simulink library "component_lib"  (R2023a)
settings: Solver=VariableStepAuto  StartTime=0.0  StopTime=10.0  RelTol=1e-3
undefined symbols (not defined in the file or in its folder): component_lib, ECCV_r, KoblenzTrier, mm, par, param_TD04, R1234yf_ph, SigIdentifier, Systems, TH0023_WP120, Thermal, V_nom
libraries: base_lib x166, $bdroot x164, simulink x2, slpidlib x1
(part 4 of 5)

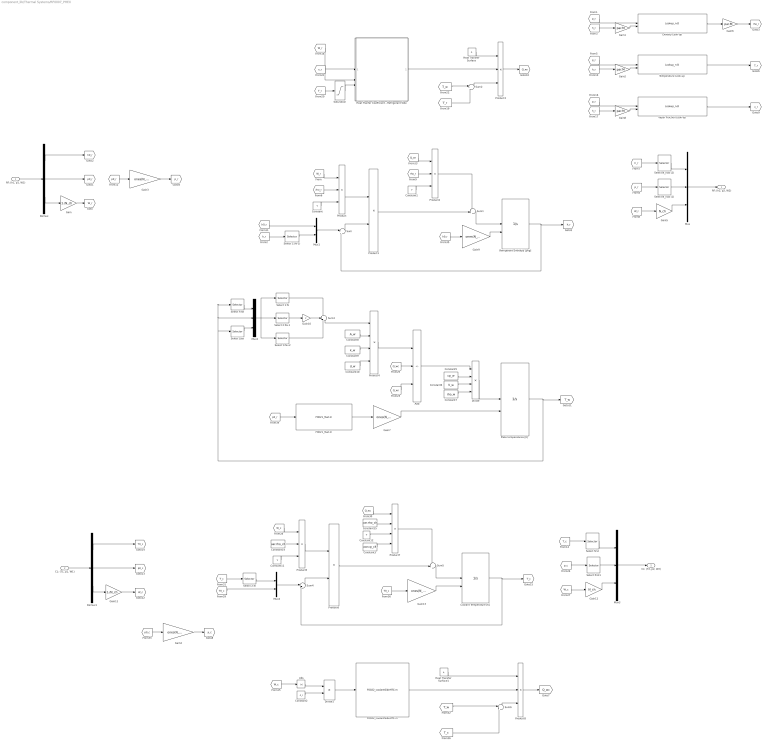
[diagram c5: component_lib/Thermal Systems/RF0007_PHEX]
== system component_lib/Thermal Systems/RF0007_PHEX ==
  "RF: (h1, p1, W1)" : Inport
  "CL: (T1, p1, W1)" : Inport  Port=2
  Abs : Abs
  Add : Sum  Inputs=+--
  Constant{,1,11..12} (4 alike) : Constant  Value=V
  Constant10 : Constant  Value=d_w
  Constant14 : Constant  Value=par.rho_clt
  Constant15 : Constant  Value=par.rho_clt
  Constant2 : Constant  Value=A_c
  Constant3 : Constant  Value=par.cp_clt
  Constant5 : Constant  Value=cp_w
  Constant6 : Constant  Value=V_w
  Constant7 : Constant  Value=rho_w
  Constant8 : Constant  Value=A_w
  Constant9 : Constant  Value=k_w
  Coolant Temperature [K] : Integrator  InitialConditionSource=external  LimitOutput=on  LowerSaturationLimit=0
  Demux : Demux  Outputs=3
  Demux1 : Demux  Outputs=3
  Density Look-up : Lookup_n-D  BreakpointsForDimension1=R1234yf_ph.p  BreakpointsForDimension2=R1234yf_ph.h  Table=R1234yf_ph.D  InternalRulePriority=Speed  RndMeth=Simplest
  Divide : Product  Inputs=*///
  Divide1 : Product  Inputs=*/
  F0021_Tsat.m : base_lib/F0021_R1234yf/F0021_Tsat.m  SystemSampleTime=-1  VariantActivationTime=update diagram  Latency=0  AutoFrameSizeCalculation=off
  F0022_coolantSideHTC.m : base_lib/F0022_heatPump/F0022_coolantSideHTC.m  SystemSampleTime=-1  VariantActivationTime=update diagram  Latency=0  AutoFrameSizeCalculation=off
  Gain : Gain  Gain=1./N_ch
  Gain{1..2,6,8} (4 alike) : Gain  Gain=par.M
  Gain10 : Gain  Gain=2
  Gain11 : Gain  Gain=1./N_ch
  Gain12 : Gain  Gain=N_ch
  Gain{3..4,7,9,13} (5 alike) : Gain  Gain=ones(N_nod,1)
  Gain5 : Gain  Gain=N_ch
  Heat Tranfer Coefficient - Refrigerant Side : Subsystem
  Heat Transfer Surface : Constant  Value=A
  Heat Transfer Surface1 : Constant  Value=A
  Mux : Mux  Inputs=3
  Mux1 : Mux  Inputs=2
  Mux2 : Mux  Inputs=3
  Mux3 : Mux  Inputs=3
  Mux4 : Mux  Inputs=2
  Plate temperatures [K] : Integrator  InitialConditionSource=external  LimitOutput=on  LowerSaturationLimit=0
  Product : Product  Inputs=*//
  Product1 : Product
  Product2 : Product  Inputs=*//
  Product3 : Product  Inputs=3
  Product4 : Product  Inputs=***/
  Product5 : Product  Inputs=*//
  Product6 : Product
  Product7 : Product  Inputs=*///
  Product8 : Product  Inputs=3
  Refrigerant Enthalpy [J/kg] : Integrator  InitialConditionSource=external  LimitOutput=on  LowerSaturationLimit=0
  Saturation : Saturate  UpperLimit=par.Tc-2  LowerLimit=0
  Select 1:(N-1) : Selector  InputPortWidth=N_nod  IndexOptions=Index vector (dialog)  Indices=[1:(N_nod-1)]  OutputSizes=1
  Select 1:N : Selector  InputPortWidth=N_nod+2  IndexOptions=Index vector (dialog)  Indices=[1:N_nod]  OutputSizes=1
  Select 2:N : Selector  InputPortWidth=N_nod  IndexOptions=Index vector (dialog)  Indices=[2:N_nod]  OutputSizes=1
  "Select 2:N+1 " : Selector  InputPortWidth=N_nod+2  IndexOptions=Index vector (dialog)  Indices=[2:(N_nod+1)]  OutputSizes=1
  Select 3:N+2 : Selector  InputPortWidth=N_nod+2  IndexOptions=Index vector (dialog)  Indices=[3:(N_nod+2)]  OutputSizes=1
  Select First : Selector  InputPortWidth=N_nod  IndexOptions=Index vector (dialog)  Indices=1  OutputSizes=1
  Select Last : Selector  InputPortWidth=N_nod  IndexOptions=Index vector (dialog)  Indices=N_nod  OutputSizes=1
  Select N_nod (1) : Selector  InputPortWidth=N_nod  IndexOptions=Index vector (dialog)  Indices=N_nod  OutputSizes=1
  Select N_nod (2) : Selector  InputPortWidth=N_nod  IndexOptions=Index vector (dialog)  Indices=N_nod  OutputSizes=1
  Select first : Selector  InputPortWidth=N_nod  IndexOptions=Index vector (dialog)  Indices=1  OutputSizes=1
  Select first1 : Selector  InputPortWidth=N_nod  IndexOptions=Index vector (dialog)  Indices=1  OutputSizes=1
  Sum{,2,4,6} (4 alike) : Sum  Inputs=|+-
  Sum1 : Sum  Inputs=++|
  Sum3 : Sum  Inputs=+-+
  Sum5 : Sum  Inputs=++|
  Temperature Look-up : Lookup_n-D  BreakpointsForDimension1=R1234yf_ph.p  BreakpointsForDimension2=R1234yf_ph.h  Table=R1234yf_ph.T  InternalRulePriority=Speed  RndMeth=Simplest
  Vapor Fraction Look-up : Lookup_n-D  BreakpointsForDimension1=R1234yf_ph.p  BreakpointsForDimension2=R1234yf_ph.h  Table=R1234yf_ph.x  InternalRulePriority=Speed  RndMeth=Simplest
  "RF: (h2, p2, W2)" : Outport
  "CL: (T2, p2, W2)" : Outport  Port=2
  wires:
  [h_r] -> Gain1/1
  Demux/2 -> [p0_r]
  "RF: (h1, p1, W1)"/1 -> Demux/1
  Mux/1 -> "RF: (h2, p2, W2)"/1
  [W_r] -> Gain5/1
  [p_r] -> Select N_nod (1)/1
  Density Look-up/1 -> Gain6/1
  Gain1/1 -> Density Look-up/2
  Gain6/1 -> [rho_r]
  Constant/1 -> Product/3
  [rho_r] -> Product/2
  [W_r] -> Product/1
  Product/1 -> Product1/1
  Sum/1 -> Product1/2
  Product1/1 -> Sum1/2
  Sum1/1 -> Refrigerant Enthalpy [J/kg]/1
  Constant1/1 -> Product2/3
  [rho_r] -> Product2/2
  Product2/1 -> Sum1/1
  Gain9/1 -> Refrigerant Enthalpy [J/kg]/2
  Refrigerant Enthalpy [J/kg]/1 -> [h_r], Sum/2
  [h_r] -> Select 1:(N-1)/1
  Select 1:(N-1)/1 -> Mux1/2
  [h0_r] -> Mux1/1
  [p_r] -> Density Look-up/1
  [p0_r] -> Gain3/1
  Gain3/1 -> [p_r]
  [h_r] -> Select N_nod (2)/1
  Select N_nod (1)/1 -> Mux/2
  Mux1/1 -> Sum/1
  [h_r] -> Gain2/1
  Gain2/1 -> Temperature Look-up/2
  [p_r] -> Temperature Look-up/1
  [Q_wr] -> Product2/1
  [h_r] -> Gain8/1
  [p_r] -> Vapor Fraction Look-up/1
  Gain8/1 -> Vapor Fraction Look-up/2
  Vapor Fraction Look-up/1 -> [x_r]
  Gain/1 -> [W_r]
  Gain7/1 -> Plate temperatures [K]/2
  Divide/1 -> Plate temperatures [K]/1
  Add/1 -> Divide/1
  Constant5/1 -> Divide/2
  Constant6/1 -> Divide/3
  Constant7/1 -> Divide/4
  [Q_wr] -> Add/3
  Plate temperatures [K]/1 -> [T_w], Select First/1, Mux2/2, Select Last/1
  Select First/1 -> Mux2/1
  Mux2/1 -> Select 3:N+2/1, "Select 2:N+1 "/1, Select 1:N/1
  Select Last/1 -> Mux2/3
  "Select 2:N+1 "/1 -> Gain10/1
  Gain10/1 -> Sum3/2
  Select 1:N/1 -> Sum3/1
  Select 3:N+2/1 -> Sum3/3
  Sum3/1 -> Product4/1
  Constant8/1 -> Product4/2
  Constant9/1 -> Product4/3
  Constant10/1 -> Product4/4
  Product4/1 -> Add/1
  [Q_wc] -> Add/2
  Gain11/1 -> [W_c]
  Demux1/2 -> [p0_c]
  "CL: (T1, p1, W1)"/1 -> Demux1/1
  [T_c] -> Select first/1
  Select first1/1 -> Mux3/2
  [W_c] -> Gain12/1
  Mux3/1 -> "CL: (T2, p2, W2)"/1
  [p_c] -> Select first1/1
  [Q_wc] -> Product7/1
  Mux4/1 -> Sum4/1
  Coolant Temperature [K]/1 -> [T_c], Sum4/2
  Product7/1 -> Sum5/1
  Gain13/1 -> Coolant Temperature [K]/2
  [T_c] -> Select 2:N/1
  Sum5/1 -> Coolant Temperature [K]/1
  Sum4/1 -> Product6/2
  Constant15/1 -> Product7/2
  Product5/1 -> Product6/1
  [W_c] -> Product5/1
  Product6/1 -> Sum5/2
  [W_r] -> Heat Tranfer Coefficient - Refrigerant Side/1(W_r [kg/s])
  [x_r] -> Heat Tranfer Coefficient - Refrigerant Side/2(x_r [-])
  [T_r] -> Saturation/1
  Heat Transfer Surface/1 -> Product3/1
  [T_w] -> Sum2/1
  Sum2/1 -> Product3/3
  [T_r] -> Sum2/2
  Product3/1 -> [Q_wr]
  Heat Tranfer Coefficient - Refrigerant Side/1(h [W/mK]) -> Product3/2
  Constant3/1 -> Product7/4
  Constant14/1 -> Product5/2
  Divide1/1 -> F0022_coolantSideHTC.m/1
  Product8/1 -> [Q_wc]
  F0022_coolantSideHTC.m/1 -> Product8/2
  Sum6/1 -> Product8/3
  [T_c] -> Sum6/2
  Temperature Look-up/1 -> [T_r]
  Gain4/1 -> [p_c]
  [p0_c] -> Gain4/1
  Saturation/1 -> Heat Tranfer Coefficient - Refrigerant Side/3(T_r [K])
  [T_w] -> Sum6/1
  Heat Transfer Surface1/1 -> Product8/1
  Constant11/1 -> Product5/3
  Constant12/1 -> Product7/3
  [T0_c] -> Mux4/2
  Select 2:N/1 -> Mux4/1
  Demux/3 -> Gain/1
  Demux/1 -> [h0_r]
  Gain5/1 -> Mux/3
  Select N_nod (2)/1 -> Mux/1
  Gain12/1 -> Mux3/3
  Select first/1 -> Mux3/1
  Demux1/3 -> Gain11/1
  Demux1/1 -> [T0_c]
  F0021_Tsat.m/1 -> Gain7/1
  [p0_r] -> F0021_Tsat.m/1
  [h0_r] -> Gain9/1
  [T0_c] -> Gain13/1
  Abs/1 -> Divide1/1
  Constant2/1 -> Divide1/2
  [W_c] -> Abs/1

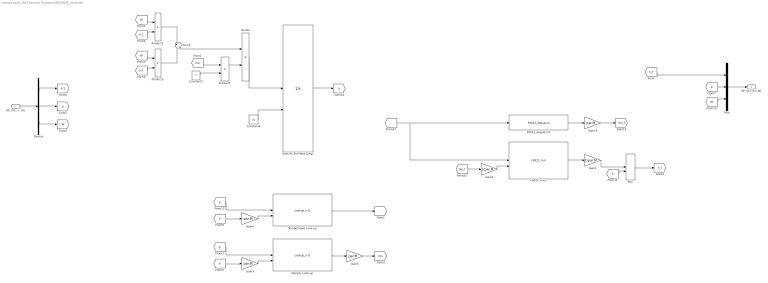
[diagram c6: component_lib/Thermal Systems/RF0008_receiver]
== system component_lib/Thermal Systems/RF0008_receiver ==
  "RF: (h1, ~, W)" : Inport
  Constant1 : Constant  Value=V
  Constant4 : Constant  Value=h0
  Demux : Demux  Outputs=3
  Density Look-up : Lookup_n-D  BreakpointsForDimension1=R1234yf_ph.p  BreakpointsForDimension2=R1234yf_ph.h  Table=R1234yf_ph.D  InternalRulePriority=Speed  RndMeth=Simplest
  Divide : Product  Inputs=*/
  F0021_dliqsat.m1 : base_lib/F0021_R1234yf/F0021_dliqsat.m  SystemSampleTime=-1  VariantActivationTime=update diagram  Latency=0  AutoFrameSizeCalculation=off
  F0021_h.m1 : base_lib/F0021_R1234yf/F0021_h.m  SystemSampleTime=-1  VariantActivationTime=update diagram  Latency=0  AutoFrameSizeCalculation=off
  Gain1 : Gain  Gain=1/par.M
  Gain{3..5,16} (4 alike) : Gain  Gain=par.M
  Gain2 : Gain  Gain=1/par.M
  Min : MinMax  Inputs=2
  Mux : Mux  Inputs=3
  Product1 : Product
  Product2 : Product
  Product3 : Product
  Specific Enthalpy [J/kg] : Integrator  InitialConditionSource=external  LimitOutput=on  LowerSaturationLimit=0
  Sum3 : Sum  Inputs=+|-
  Temperature Look-up : Lookup_n-D  BreakpointsForDimension1=R1234yf_ph.p  BreakpointsForDimension2=R1234yf_ph.h  Table=R1234yf_ph.T  InternalRulePriority=Speed  RndMeth=Simplest
  "RF: (h2, p2, W)" : Outport
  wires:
  F0021_h.m1/1 -> Gain1/1
  Gain2/1 -> F0021_h.m1/2
  [rho_f] -> Gain2/1
  [T] -> F0021_dliqsat.m1/1, F0021_h.m1/1
  F0021_dliqsat.m1/1 -> Gain16/1
  Gain16/1 -> [rho_f]
  [h_1] -> Product2/2
  [W] -> Product2/1
  Product2/1 -> Sum3/1
  [h_f] -> Product3/2
  Product3/1 -> Sum3/2
  [W] -> Product3/1
  Specific Enthalpy [J/kg]/1 -> [h]
  [h] -> Gain4/1
  Temperature Look-up/1 -> [T]
  Gain4/1 -> Temperature Look-up/2
  [p] -> Temperature Look-up/1
  Constant1/1 -> Product1/2
  [rho] -> Product1/1
  Density Look-up/1 -> Gain5/1
  Gain3/1 -> Density Look-up/2
  [p] -> Density Look-up/1
  [h] -> Gain3/1
  Gain5/1 -> [rho]
  Divide/1 -> Specific Enthalpy [J/kg]/1
  Sum3/1 -> Divide/1
  Product1/1 -> Divide/2
  Constant4/1 -> Specific Enthalpy [J/kg]/2
  Mux/1 -> "RF: (h2, p2, W)"/1
  [p] -> Mux/2
  [W] -> Mux/3
  "RF: (h1, ~, W)"/1 -> Demux/1
  Demux/1 -> [h_1]
  Demux/3 -> [W]
  [h_f] -> Mux/1
  Demux/2 -> [p]
  Min/1 -> [h_f]
  Gain1/1 -> Min/1
  [h] -> Min/2

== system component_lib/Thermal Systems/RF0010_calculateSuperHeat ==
  "RF: (h, p, W)" : Inport
  Demux : Demux  Outputs=3
  F0021_Tsat.m : base_lib/F0021_R1234yf/F0021_Tsat.m  SystemSampleTime=-1  VariantActivationTime=update diagram  Latency=0  AutoFrameSizeCalculation=off
  Gain2 : Gain  Gain=par.M
  Saturation : Saturate  UpperLimit=inf  LowerLimit=0
  Sum : Sum  Inputs=|+-
  Temperature Look-up : Lookup_n-D  BreakpointsForDimension1=R1234yf_ph.p  BreakpointsForDimension2=R1234yf_ph.h  Table=R1234yf_ph.T  InternalRulePriority=Speed  RndMeth=Simplest
  T_sup [K] : Outport
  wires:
  Demux/2 -> [p]
  Gain2/1 -> Temperature Look-up/2
  [p] -> F0021_Tsat.m/1, Temperature Look-up/1
  [h] -> Gain2/1
  Temperature Look-up/1 -> Sum/1
  F0021_Tsat.m/1 -> Sum/2
  Sum/1 -> Saturation/1
  Saturation/1 -> T_sup [K]/1
  "RF: (h, p, W)"/1 -> Demux/1
  Demux/1 -> [h]
  Demux/3 -> [W]

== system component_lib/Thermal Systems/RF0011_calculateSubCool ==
  "RF: (h, p, W)" : Inport
  Demux : Demux  Outputs=3
  F0021_Tsat.m : base_lib/F0021_R1234yf/F0021_Tsat.m  SystemSampleTime=-1  VariantActivationTime=update diagram  Latency=0  AutoFrameSizeCalculation=off
  Gain2 : Gain  Gain=par.M
  Saturation : Saturate  UpperLimit=inf  LowerLimit=0
  Sum : Sum  Inputs=|+-
  Temperature Look-up : Lookup_n-D  BreakpointsForDimension1=R1234yf_ph.p  BreakpointsForDimension2=R1234yf_ph.h  Table=R1234yf_ph.T  InternalRulePriority=Speed  RndMeth=Simplest
  T_sub [K] : Outport
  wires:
  "RF: (h, p, W)"/1 -> Demux/1
  Demux/2 -> [p]
  Gain2/1 -> Temperature Look-up/2
  [p] -> F0021_Tsat.m/1, Temperature Look-up/1
  [h] -> Gain2/1
  Sum/1 -> Saturation/1
  F0021_Tsat.m/1 -> Sum/1
  Temperature Look-up/1 -> Sum/2
  Saturation/1 -> T_sub [K]/1
  Demux/1 -> [h]
  Demux/3 -> [W]

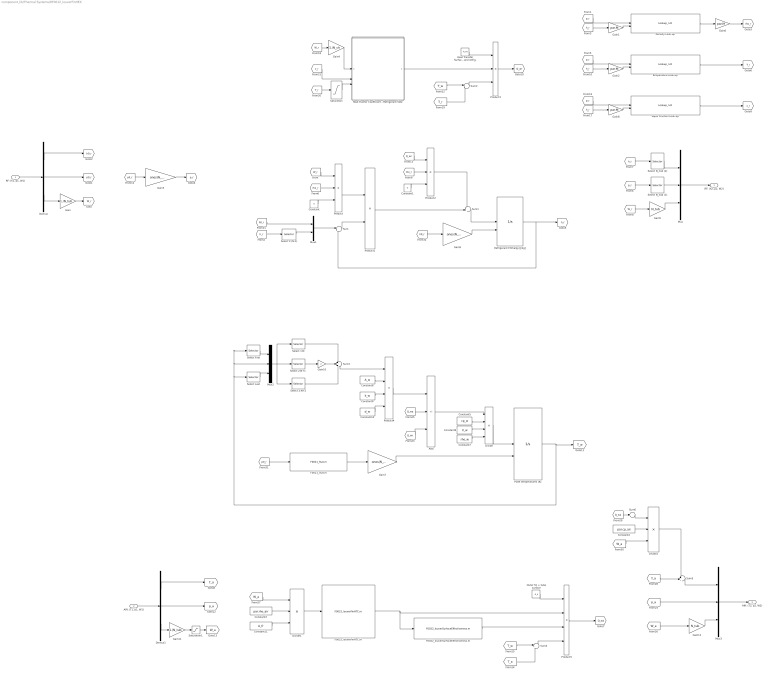
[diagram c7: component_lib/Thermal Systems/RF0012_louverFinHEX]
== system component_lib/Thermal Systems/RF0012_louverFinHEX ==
  "RF: (h1, p1, W1)" : Inport
  "AIR: (T1, p1, W1)" : Inport  Port=2
  Add : Sum  Inputs=+--
  Constant : Constant  Value=V
  Constant1 : Constant  Value=V
  Constant10 : Constant  Value=d_w
  Constant11 : Constant  Value=A_fr
  Constant2 : Constant  Value=par.cp_air
  Constant3 : Constant  Value=par.rho_air
  Constant5 : Constant  Value=cp_w
  Constant6 : Constant  Value=V_w
  Constant7 : Constant  Value=rho_w
  Constant8 : Constant  Value=A_w
  Constant9 : Constant  Value=k_w
  Demux : Demux  Outputs=3
  Demux1 : Demux  Outputs=3
  Density Look-up : Lookup_n-D  BreakpointsForDimension1=R1234yf_ph.p  BreakpointsForDimension2=R1234yf_ph.h  Table=R1234yf_ph.D  InternalRulePriority=Speed  RndMeth=Simplest
  Divide : Product  Inputs=*///
  Divide1 : Product  Inputs=*//
  Divide2 : Product  Inputs=*//
  F0021_Tsat.m : base_lib/F0021_R1234yf/F0021_Tsat.m  SystemSampleTime=-1  VariantActivationTime=update diagram  Latency=0  AutoFrameSizeCalculation=off
  F0022_louverFinHTC.m : base_lib/F0022_heatPump/F0022_louverFinHTC.m  SystemSampleTime=-1  VariantActivationTime=update diagram  Latency=0  AutoFrameSizeCalculation=off
  F0022_louverSurfaceEffectiveness.m : base_lib/F0022_heatPump/F0022_louverSurfaceEffectiveness.m  SystemSampleTime=-1  VariantActivationTime=update diagram  Latency=0  AutoFrameSizeCalculation=off
  Gain : Gain  Gain=1./N_tub
  Gain{1..2,6,8} (4 alike) : Gain  Gain=par.M
  Gain10 : Gain  Gain=2
  Gain11 : Gain  Gain=1./N_tub
  Gain12 : Gain  Gain=N_tub
  Gain3 : Gain  Gain=ones(N_nod,1)
  Gain4 : Gain  Gain=1./N_ch
  Gain5 : Gain  Gain=N_tub
  Gain7 : Gain  Gain=ones(N_nod,1)
  Gain9 : Gain  Gain=ones(N_nod,1)
  Heat Tranfer Coefficient - Refrigerant Side : Subsystem
  Heat Transfer Surface between wall and refrig. : Constant  Value=A_wr
  Mux : Mux  Inputs=3
  Mux1 : Mux  Inputs=2
  Mux2 : Mux  Inputs=3
  Mux3 : Mux  Inputs=3
  Outer fin + tube surface : Constant  Value=A_o
  Plate temperatures [K] : Integrator  InitialConditionSource=external  LimitOutput=on  LowerSaturationLimit=0
  Product : Product  Inputs=*//
  Product1 : Product
  Product2 : Product  Inputs=*//
  Product3 : Product  Inputs=3
  Product4 : Product  Inputs=***/
  Product5 : Product  Inputs=4
  Refrigerant Enthalpy [J/kg] : Integrator  InitialConditionSource=external  LimitOutput=on  LowerSaturationLimit=0
  Saturation : Saturate  UpperLimit=par.Tc-2  LowerLimit=0
  Saturation1 : Saturate  UpperLimit=inf  LowerLimit=1e-5
  Select 1:(N-1) : Selector  InputPortWidth=N_nod  IndexOptions=Index vector (dialog)  Indices=[1:(N_nod-1)]  OutputSizes=1
  Select 1:N : Selector  InputPortWidth=N_nod+2  IndexOptions=Index vector (dialog)  Indices=[1:N_nod]  OutputSizes=1
  "Select 2:N+1 " : Selector  InputPortWidth=N_nod+2  IndexOptions=Index vector (dialog)  Indices=[2:(N_nod+1)]  OutputSizes=1
  Select 3:N+2 : Selector  InputPortWidth=N_nod+2  IndexOptions=Index vector (dialog)  Indices=[3:(N_nod+2)]  OutputSizes=1
  Select First : Selector  InputPortWidth=N_nod  IndexOptions=Index vector (dialog)  Indices=1  OutputSizes=1
  Select Last : Selector  InputPortWidth=N_nod  IndexOptions=Index vector (dialog)  Indices=N_nod  OutputSizes=1
  Select N_nod (1) : Selector  InputPortWidth=N_nod  IndexOptions=Index vector (dialog)  Indices=N_nod  OutputSizes=1
  Select N_nod (2) : Selector  InputPortWidth=N_nod  IndexOptions=Index vector (dialog)  Indices=N_nod  OutputSizes=1
  Sum : Sum  Inputs=|+-
  Sum1 : Sum  Inputs=++|
  Sum2 : Sum  Inputs=|+-
  Sum3 : Sum  Inputs=+-+
  Sum4 : Sum  Inputs=|+-
  Sum5 : Sum  Inputs=++|
  Sum6 : Sum  Inputs=+
  Temperature Look-up : Lookup_n-D  BreakpointsForDimension1=R1234yf_ph.p  BreakpointsForDimension2=R1234yf_ph.h  Table=R1234yf_ph.T  InternalRulePriority=Speed  RndMeth=Simplest
  Vapor Fraction Look-up : Lookup_n-D  BreakpointsForDimension1=R1234yf_ph.p  BreakpointsForDimension2=R1234yf_ph.h  Table=R1234yf_ph.x  InternalRulePriority=Speed  RndMeth=Simplest
  "RF: (h2, p2, W2)" : Outport
  "AIR: (T2, p2, W2)" : Outport  Port=2
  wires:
  Select N_nod (2)/1 -> Mux/1
  Gain5/1 -> Mux/3
  Demux/1 -> [h0_r]
  Demux/3 -> Gain/1
  Saturation/1 -> Heat Tranfer Coefficient - Refrigerant Side/3(T_r [K])
  Temperature Look-up/1 -> [T_r]
  Heat Tranfer Coefficient - Refrigerant Side/1(h [W/mK]) -> Product3/2
  Product3/1 -> [Q_wr]
  [T_r] -> Sum2/2
  Sum2/1 -> Product3/3
  [T_w] -> Sum2/1
  Heat Transfer Surface between wall and refrig./1 -> Product3/1
  [T_r] -> Saturation/1
  [x_r] -> Heat Tranfer Coefficient - Refrigerant Side/2(x_r [-])
  Mux3/1 -> "AIR: (T2, p2, W2)"/1
  "AIR: (T1, p1, W1)"/1 -> Demux1/1
  [Q_wa] -> Add/2
  Product4/1 -> Add/1
  Constant10/1 -> Product4/4
  Constant8/1 -> Product4/2
  Sum3/1 -> Product4/1
  Select 3:N+2/1 -> Sum3/3
  Select 1:N/1 -> Sum3/1
  Gain10/1 -> Sum3/2
  "Select 2:N+1 "/1 -> Gain10/1
  Select Last/1 -> Mux2/3
  Mux2/1 -> Select 1:N/1, "Select 2:N+1 "/1, Select 3:N+2/1
  Select First/1 -> Mux2/1
  Plate temperatures [K]/1 -> Mux2/2, Select First/1, Select Last/1, [T_w]
  [Q_wr] -> Add/3
  Constant7/1 -> Divide/4
  Constant6/1 -> Divide/3
  Constant5/1 -> Divide/2
  Add/1 -> Divide/1
  Divide/1 -> Plate temperatures [K]/1
  Gain7/1 -> Plate temperatures [K]/2
  Gain/1 -> [W_r]
  Vapor Fraction Look-up/1 -> [x_r]
  Gain8/1 -> Vapor Fraction Look-up/2
  [p_r] -> Vapor Fraction Look-up/1
  [h_r] -> Gain8/1
  [Q_wr] -> Product2/1
  [p_r] -> Temperature Look-up/1
  Gain2/1 -> Temperature Look-up/2
  [h_r] -> Gain2/1
  Mux1/1 -> Sum/1
  Select N_nod (1)/1 -> Mux/2
  [h_r] -> Select N_nod (2)/1
  Gain3/1 -> [p_r]
  [p0_r] -> Gain3/1
  [p_r] -> Density Look-up/1
  [h0_r] -> Mux1/1
  Select 1:(N-1)/1 -> Mux1/2
  [h_r] -> Select 1:(N-1)/1
  Refrigerant Enthalpy [J/kg]/1 -> Sum/2, [h_r]
  Gain9/1 -> Refrigerant Enthalpy [J/kg]/2
  Product2/1 -> Sum1/1
  [rho_r] -> Product2/2
  Constant1/1 -> Product2/3
  Sum1/1 -> Refrigerant Enthalpy [J/kg]/1
  Product1/1 -> Sum1/2
  Sum/1 -> Product1/2
  Product/1 -> Product1/1
  [W_r] -> Product/1
  [rho_r] -> Product/2
  Constant/1 -> Product/3
  Gain6/1 -> [rho_r]
  Gain1/1 -> Density Look-up/2
  Density Look-up/1 -> Gain6/1
  [p_r] -> Select N_nod (1)/1
  [W_r] -> Gain5/1
  Mux/1 -> "RF: (h2, p2, W2)"/1
  "RF: (h1, p1, W1)"/1 -> Demux/1
  Demux/2 -> [p0_r]
  [h_r] -> Gain1/1
  F0022_louverFinHTC.m/1 -> Product5/2, F0022_louverSurfaceEffectiveness.m/1
  Divide1/1 -> F0022_louverFinHTC.m/1
  Constant3/1 -> Divide1/2
  Constant11/1 -> Divide1/3
  Product5/1 -> [Q_wa]
  [T_w] -> Sum4/1
  Outer fin + tube surface/1 -> Product5/1
  [T_a] -> Sum4/2
  Sum4/1 -> Product5/4
  F0022_louverSurfaceEffectiveness.m/1 -> Product5/3
  Demux1/1 -> [T_a]
  Demux1/2 -> [p_a]
  [p_a] -> Mux3/2
  Demux1/3 -> Gain11/1
  [W_a] -> Divide1/1
  [W_r] -> Gain4/1
  Gain4/1 -> Heat Tranfer Coefficient - Refrigerant Side/1(W_r [kg/s])
  [p0_r] -> F0021_Tsat.m/1
  F0021_Tsat.m/1 -> Gain7/1
  [h0_r] -> Gain9/1
  Constant9/1 -> Product4/3
  Gain12/1 -> Mux3/3
  Gain11/1 -> Saturation1/1
  [W_a] -> Gain12/1
  [T_a] -> Sum5/2
  Sum5/1 -> Mux3/1
  [Q_wa] -> Sum6/1
  Sum6/1 -> Divide2/1
  Constant2/1 -> Divide2/2
  [W_a] -> Divide2/3
  Divide2/1 -> Sum5/1
  Saturation1/1 -> [W_a]

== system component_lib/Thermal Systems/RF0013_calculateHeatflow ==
  "RF: (h1, p1, W1)" : Inport
  "RF: (h2, p2, W2)" : Inport  Port=2
  Demux : Demux  Outputs=3
  Demux1 : Demux  Outputs=3
  Product : Product
  Product1 : Product
  Sum : Sum  Inputs=|+-
  Terminator : Terminator
  Terminator1 : Terminator
  Q [J/s] : Outport
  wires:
  "RF: (h1, p1, W1)"/1 -> Demux/1
  "RF: (h2, p2, W2)"/1 -> Demux1/1
  Sum/1 -> Q [J/s]/1
  Demux/2 -> Terminator/1
  Demux1/2 -> Terminator1/1
  Demux/1 -> Product/1
  Demux/3 -> Product/2
  Demux1/1 -> Product1/1
  Demux1/3 -> Product1/2
  Product1/1 -> Sum/1
  Product/1 -> Sum/2

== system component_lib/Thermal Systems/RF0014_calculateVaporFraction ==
  "RF: (h, p, W)" : Inport
  Demux : Demux  Outputs=3
  Gain2 : Gain  Gain=par.M
  Vapor Fraction Look-up : Lookup_n-D  BreakpointsForDimension1=R1234yf_ph.p  BreakpointsForDimension2=R1234yf_ph.h  Table=R1234yf_ph.x  InternalRulePriority=Speed  RndMeth=Simplest
  x [-] : Outport
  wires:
  Demux/2 -> [p]
  Gain2/1 -> Vapor Fraction Look-up/2
  [p] -> Vapor Fraction Look-up/1
  [h] -> Gain2/1
  Vapor Fraction Look-up/1 -> x [-]/1
  "RF: (h, p, W)"/1 -> Demux/1
  Demux/1 -> [h]
  Demux/3 -> [W]

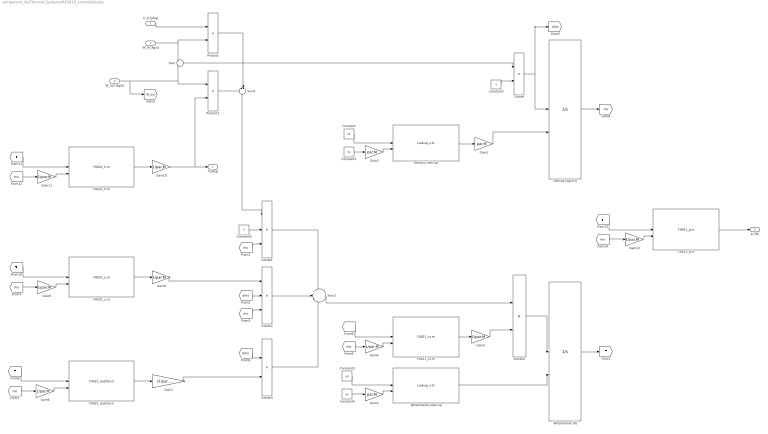
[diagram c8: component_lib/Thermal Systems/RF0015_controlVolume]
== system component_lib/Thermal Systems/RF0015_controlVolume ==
  h_in [J/kg] : Inport
  W_in [kg/s] : Inport  Port=2
  W_out [kg/s] : Inport  Port=3
  Constant : Constant  Value=p0
  Constant1 : Constant  Value=h0
  Constant2 : Constant  Value=V
  Constant3 : Constant  Value=p0
  Constant4 : Constant  Value=h0
  Constant5 : Constant  Value=V
  Density Look-up : Lookup_n-D  BreakpointsForDimension1=R1234yf_ph.p  BreakpointsForDimension2=R1234yf_ph.h  Table=R1234yf_ph.D  InternalRulePriority=Speed  RndMeth=Simplest
  Density [kg/m3] : Integrator  InitialConditionSource=external  LimitOutput=on  LowerSaturationLimit=0
  Divide : Product  Inputs=*/
  Divide1 : Product  Inputs=*//
  Divide2 : Product  Inputs=**/
  Divide3 : Product  Inputs=**
  Divide4 : Product  Inputs=*/
  F0021_cv.m : base_lib/F0021_R1234yf/F0021_cv.m  SystemSampleTime=-1  VariantActivationTime=update diagram  Latency=0  AutoFrameSizeCalculation=off
  F0021_dudrho.m : base_lib/F0021_R1234yf/F0021_dudrho.m  SystemSampleTime=-1  VariantActivationTime=update diagram  Latency=0  AutoFrameSizeCalculation=off
  F0021_h.m : base_lib/F0021_R1234yf/F0021_h.m  SystemSampleTime=-1  VariantActivationTime=update diagram  Latency=0  AutoFrameSizeCalculation=off
  F0021_p.m : base_lib/F0021_R1234yf/F0021_p.m  SystemSampleTime=-1  VariantActivationTime=update diagram  Latency=0  AutoFrameSizeCalculation=off
  F0021_u.m : base_lib/F0021_R1234yf/F0021_u.m  SystemSampleTime=-1  VariantActivationTime=update diagram  Latency=0  AutoFrameSizeCalculation=off
  Gain1 : Gain  Gain=par.M
  Gain{4..6,8..12} (8 alike) : Gain  Gain=1/par.M
  Gain2 : Gain  Gain=par.M
  Gain3 : Gain  Gain=par.M
  Gain7 : Gain  Gain=(1/par.M).^2
  Product : Product
  Product1 : Product
  Sum : Sum  Inputs=+|-
  Sum1 : Sum  Inputs=-+|
  Sum2 : Sum  Inputs=+--
  Temperature Look-up : Lookup_n-D  BreakpointsForDimension1=R1234yf_ph.p  BreakpointsForDimension2=R1234yf_ph.h  Table=R1234yf_ph.T  InternalRulePriority=Speed  RndMeth=Simplest
  Temperature [K] : Integrator  InitialConditionSource=external  LimitOutput=on  LowerSaturationLimit=0
  h [J/kg] : Outport
  p [Pa] : Outport  Port=2
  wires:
  Density Look-up/1 -> Gain1/1
  Gain1/1 -> Density [kg/m3]/2
  Constant/1 -> Density Look-up/1
  Gain3/1 -> Density Look-up/2
  Constant1/1 -> Gain3/1
  Divide/1 -> Density [kg/m3]/1, [drho]
  Constant2/1 -> Divide/2
  Density [kg/m3]/1 -> [rho]
  Sum/1 -> Divide/1
  W_out [kg/s]/1 -> [W_out], Product1/1, Sum/2
  Temperature Look-up/1 -> Temperature [K]/2
  Gain2/1 -> Temperature Look-up/2
  Constant4/1 -> Gain2/1
  Constant3/1 -> Temperature Look-up/1
  Temperature [K]/1 -> [T]
  W_in [kg/s]/1 -> Product/2, Sum/1
  h_in [J/kg]/1 -> Product/1
  Gain10/1 -> h [J/kg]/1, Product1/2
  Product/1 -> Sum1/2
  Product1/1 -> Sum1/1
  Sum1/1 -> Divide1/1
  Constant5/1 -> Divide1/2
  [rho] -> Divide1/3
  [rho] -> Divide2/3
  [drho] -> Divide2/2
  Gain9/1 -> Divide2/1
  [rho] -> Gain4/1
  Gain4/1 -> F0021_cv.m/2
  F0021_cv.m/1 -> Gain5/1
  [T] -> F0021_cv.m/1
  Divide4/1 -> Temperature [K]/1
  Gain5/1 -> Divide4/2
  Sum2/1 -> Divide4/1
  Divide1/1 -> Sum2/1
  Divide2/1 -> Sum2/2
  Divide3/1 -> Sum2/3
  [rho] -> Gain6/1
  Gain6/1 -> F0021_dudrho.m/2
  [T] -> F0021_dudrho.m/1
  [drho] -> Divide3/1
  F0021_dudrho.m/1 -> Gain7/1
  Gain7/1 -> Divide3/2
  [T] -> F0021_u.m/1
  [rho] -> Gain8/1
  Gain8/1 -> F0021_u.m/2
  F0021_u.m/1 -> Gain9/1
  F0021_h.m/1 -> Gain10/1
  [rho] -> Gain11/1
  Gain11/1 -> F0021_h.m/2
  [T] -> F0021_h.m/1
  F0021_p.m/1 -> p [Pa]/1
  [rho] -> Gain12/1
  Gain12/1 -> F0021_p.m/2
  [T] -> F0021_p.m/1

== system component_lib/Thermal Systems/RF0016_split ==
  "RF A: (h, p, W)" : Inport
  split [-] : Inport  Port=2
  Constant : Constant
  Demux : Demux  Outputs=3
  Mux : Mux  Inputs=3
  Mux1 : Mux  Inputs=3
  Product : Product
  Product1 : Product
  Sum : Sum  Inputs=-+|
  "RF B: (h, p, Wb)" : Outport
  "RF C: (h, p, Wc)" : Outport  Port=2
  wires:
  "RF A: (h, p, W)"/1 -> Demux/1
  Mux/1 -> "RF B: (h, p, Wb)"/1
  Mux1/1 -> "RF C: (h, p, Wc)"/1
  Demux/3 -> [W]
  Demux/2 -> [p]
  Demux/1 -> [h]
  split [-]/1 -> Sum/1, Product/2
  [W] -> Product/1
  Constant/1 -> Sum/2
  Sum/1 -> Product1/2
  [W] -> Product1/1
  Product/1 -> Mux/3
  [p] -> Mux/2
  [p] -> Mux1/2
  [h] -> Mux/1
  [h] -> Mux1/1
  Product1/1 -> Mux1/3

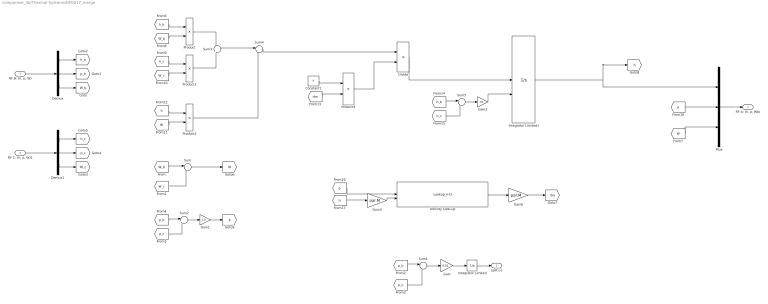
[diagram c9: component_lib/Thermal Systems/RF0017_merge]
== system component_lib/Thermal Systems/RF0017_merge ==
  "RF B: (h, p, W)" : Inport
  "RF C: (h, p, W)1" : Inport  Port=2
  Constant1 : Constant  Value=V
  Demux : Demux  Outputs=3
  Demux1 : Demux  Outputs=3
  Density Look-up : Lookup_n-D  BreakpointsForDimension1=R1234yf_ph.p  BreakpointsForDimension2=R1234yf_ph.h  Table=R1234yf_ph.D  InternalRulePriority=Speed  RndMeth=Simplest
  Divide : Product  Inputs=*/
  Gain : Gain  Gain=0.01
  Gain1 : Gain  Gain=1/2
  Gain2 : Gain  Gain=1/2
  Gain3 : Gain  Gain=par.M
  Gain6 : Gain  Gain=par.M
  Integrator Limited : Integrator  InitialCondition=0.5  LimitOutput=on  UpperSaturationLimit=1  LowerSaturationLimit=0
  Integrator Limited1 : Integrator  InitialConditionSource=external  InitialCondition=0.5  LimitOutput=on  LowerSaturationLimit=0
  Mux : Mux  Inputs=3
  Product{,1..2,4} (4 alike) : Product
  Sum : Sum  Inputs=|++
  Sum1 : Sum  Inputs=|+-
  Sum2 : Sum  Inputs=|++
  Sum3 : Sum  Inputs=+|+
  Sum4 : Sum  Inputs=|+-
  Sum5 : Sum  Inputs=|++
  "RF A: (h, p, Wb)" : Outport
  split [-] : Outport  Port=2
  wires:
  "RF B: (h, p, W)"/1 -> Demux/1
  Mux/1 -> "RF A: (h, p, Wb)"/1
  Demux/3 -> [W_b]
  Demux/2 -> [p_b]
  Demux/1 -> [h_b]
  Sum2/1 -> Gain1/1
  Demux1/1 -> [h_c]
  Demux1/3 -> [W_c]
  Demux1/2 -> [p_c]
  "RF C: (h, p, W)1"/1 -> Demux1/1
  [W_b] -> Sum/1
  [W_c] -> Sum/2
  [p_c] -> Sum1/2
  [p_b] -> Sum1/1
  Gain/1 -> Integrator Limited/1
  Sum1/1 -> Gain/1
  Integrator Limited/1 -> split [-]/1
  [p_b] -> Sum2/1
  [p_c] -> Sum2/2
  [h_b] -> Product/1
  [W_b] -> Product/2
  [W_c] -> Product1/2
  [h_c] -> Product1/1
  Product/1 -> Sum3/1
  Product1/1 -> Sum3/2
  Sum3/1 -> Sum4/1
  Sum/1 -> [W]
  [h] -> Product2/1
  [W] -> Product2/2
  [W] -> Mux/3
  Product2/1 -> Sum4/2
  Constant1/1 -> Product4/1
  [rho] -> Product4/2
  [h_b] -> Sum5/1
  [h_c] -> Sum5/2
  Sum5/1 -> Gain2/1
  Gain2/1 -> Integrator Limited1/2
  Divide/1 -> Integrator Limited1/1
  Sum4/1 -> Divide/1
  Product4/1 -> Divide/2
  Integrator Limited1/1 -> [h], Mux/1
  Density Look-up/1 -> Gain6/1
  [h] -> Gain3/1
  Gain3/1 -> Density Look-up/2
  Gain6/1 -> [rho]
  [p] -> Density Look-up/1
  Gain1/1 -> [p]
  [p] -> Mux/2

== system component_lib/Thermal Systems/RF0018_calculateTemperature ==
  "RF: (h, p, W)" : Inport
  Demux : Demux  Outputs=3
  Gain2 : Gain  Gain=par.M
  Temperature Look-up : Lookup_n-D  BreakpointsForDimension1=R1234yf_ph.p  BreakpointsForDimension2=R1234yf_ph.h  Table=R1234yf_ph.T  InternalRulePriority=Speed  RndMeth=Simplest
  T [K] : Outport
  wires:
  "RF: (h, p, W)"/1 -> Demux/1
  Demux/2 -> [p]
  Gain2/1 -> Temperature Look-up/2
  [p] -> Temperature Look-up/1
  [h] -> Gain2/1
  Temperature Look-up/1 -> T [K]/1
  Demux/1 -> [h]
  Demux/3 -> [W]

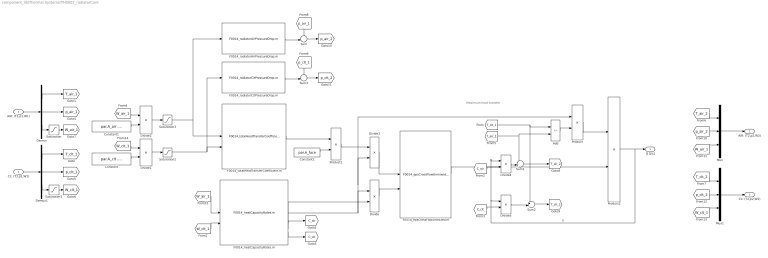
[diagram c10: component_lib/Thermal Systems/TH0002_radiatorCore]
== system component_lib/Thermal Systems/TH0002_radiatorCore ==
  note: Maximum heat transfer
  AIR: (T1,p1,W1) : Inport
  CL: (T1,p1,W1) : Inport  Port=2
  Add : Sum  Inputs=+-
  Constant : Constant  Value=par.A_clt .* par.rho_clt
  Constant1 : Constant  Value=par.A_air .* par.rho_air
  Constant2 : Constant  Value=par.A_face
  Demux : Demux  Outputs=3
  Demux1 : Demux  Outputs=3
  Divide{,1..5} (6 alike) : Product  Inputs=*/
  F0014_epsCrossFlowUnmixed.m : base_lib/F0014_titanXradiator/F0014_epsCrossFlowUnmixed.m  SystemSampleTime=-1  VariantActivationTime=update diagram  Latency=0  AutoFrameSizeCalculation=off
  F0014_heatCapacityRates.m : base_lib/F0014_titanXradiator/F0014_heatCapacityRates.m  SystemSampleTime=-1  VariantActivationTime=update diagram  Latency=0  AutoFrameSizeCalculation=off
  F0014_radiatorAirPressureDrop.m : base_lib/F0014_titanXradiator/F0014_radiatorAirPressureDrop.m  SystemSampleTime=-1  VariantActivationTime=update diagram  Latency=0  AutoFrameSizeCalculation=off
  F0014_radiatorCltPressureDrop.m : base_lib/F0014_titanXradiator/F0014_radiatorCltPressureDrop.m  SystemSampleTime=-1  VariantActivationTime=update diagram  Latency=0  AutoFrameSizeCalculation=off
  F0014_totalHeatTransferCoefficient.m : base_lib/F0014_titanXradiator/F0014_totalHeatTransferCoefficient.m  SystemSampleTime=-1  VariantActivationTime=update diagram  Latency=0  AutoFrameSizeCalculation=off
  Mux : Mux  Inputs=3
  Mux1 : Mux  Inputs=3
  Product : Product
  Product1 : Product
  Product2 : Product
  Saturation : Saturate  UpperLimit=inf  LowerLimit=1e-5
  Saturation1 : Saturate  UpperLimit=inf  LowerLimit=1e-5
  Saturation2 : Saturate  UpperLimit=inf  LowerLimit=1e-3
  Saturation3 : Saturate  UpperLimit=inf  LowerLimit=1e-3
  Sum : Sum  Inputs=+-|
  Sum1 : Sum  Inputs=++|
  Sum2 : Sum  Inputs=+-|
  Sum3 : Sum  Inputs=+-|
  Q [J/s] : Outport
  AIR: (T2,p2,W2) : Outport  Port=2
  CL: (T2,p2,W2) : Outport  Port=3
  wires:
  F0014_heatCapacityRates.m/2 -> Divide/2
  F0014_heatCapacityRates.m/1 -> Product/1, Divide3/2, Divide/1
  Divide/1 -> F0014_epsCrossFlowUnmixed.m/2
  Constant/1 -> Divide1/2
  Divide1/1 -> Saturation2/1
  [W_air_1] -> Divide2/1
  Constant1/1 -> Divide2/2
  Divide2/1 -> Saturation3/1
  F0014_totalHeatTransferCoefficient.m/1 -> Product1/1
  Constant2/1 -> Product1/2
  Product1/1 -> Divide3/1
  Divide3/1 -> F0014_epsCrossFlowUnmixed.m/1
  F0014_epsCrossFlowUnmixed.m/1 -> Product2/2
  Add/1 -> Product/2
  Product2/1 -> Q [J/s]/1, Divide4/1, Divide5/1  "Q"
  [T_clt_1] -> Sum2/1, Add/1
  Product/1 -> Product2/1
  F0014_heatCapacityRates.m/3 -> [C_air]
  F0014_heatCapacityRates.m/4 -> [C_clt]
  [T_air_1] -> Add/2, Sum1/1
  Divide4/1 -> Sum1/2
  [C_air] -> Divide4/2
  [C_clt] -> Divide5/2
  Divide5/1 -> Sum2/2
  AIR: (T1,p1,W1)/1 -> Demux/1
  CL: (T1,p1,W1)/1 -> Demux1/1
  Demux1/1 -> [T_clt_1]
  Demux/1 -> [T_air_1]
  Demux/2 -> [p_air_1]
  Demux1/2 -> [p_clt_1]
  Sum1/1 -> [T_air_2]
  Sum2/1 -> [T_clt_2]
  Mux/1 -> AIR: (T2,p2,W2)/1
  [p_air_1] -> Sum/1
  F0014_radiatorAirPressureDrop.m/1 -> Sum/2
  Sum/1 -> [p_air_2]
  Sum3/1 -> [p_clt_2]
  F0014_radiatorCltPressureDrop.m/1 -> Sum3/2
  [p_clt_1] -> Sum3/1
  [T_clt_2] -> Mux1/1
  [T_air_2] -> Mux/1
  [p_air_2] -> Mux/2
  [W_air_1] -> Mux/3
  [p_clt_2] -> Mux1/2
  [W_clt_1] -> Mux1/3
  Mux1/1 -> CL: (T2,p2,W2)/1
  Demux1/3 -> Saturation1/1
  Saturation1/1 -> [W_clt_1]
  Demux/3 -> Saturation/1
  Saturation/1 -> [W_air_1]
  [W_clt_1] -> F0014_heatCapacityRates.m/2
  [W_clt_1] -> Divide1/1
  [W_air_1] -> F0014_heatCapacityRates.m/1
  Saturation2/1 -> F0014_radiatorCltPressureDrop.m/1, F0014_totalHeatTransferCoefficient.m/2
  Saturation3/1 -> F0014_radiatorAirPressureDrop.m/1, F0014_totalHeatTransferCoefficient.m/1

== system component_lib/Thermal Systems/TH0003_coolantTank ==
  CL: (T1,p1,W1) : Inport
  Coolant density : Constant  Value=par.rho_clt
  Coolant density1 : Constant  Value=par.rho_clt
  Demux1 : Demux  Outputs=3
  Divide : Product  Inputs=*/
  F0014_tankPressureDrop.m : base_lib/F0014_titanXradiator/F0014_tankPressureDrop.m  SystemSampleTime=-1  VariantActivationTime=update diagram  Latency=0  AutoFrameSizeCalculation=off
  Integrator : Integrator  InitialCondition=T_0
  Mixing/Mass factor - empirical : Gain  Gain=3
  Mux1 : Mux  Inputs=3
  Product : Product
  Product1 : Product
  Product3 : Product  Inputs=*/
  Product5 : Product  Inputs=*/
  Subtract : Sum  Inputs=+-
  Sum : Sum  Inputs=|+-
  Tank volume : Constant  Value=par.V
  connector inlet area : Constant  Value=par.A_con
  CL: (T2,p2,W2) : Outport
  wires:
  CL: (T1,p1,W1)/1 -> Demux1/1
  Demux1/3 -> [W_clt_1]
  Demux1/1 -> [T_clt_1]
  Demux1/2 -> [p_clt_1]
  Mux1/1 -> CL: (T2,p2,W2)/1
  [p_clt_2] -> Mux1/2
  [W_clt_1] -> Mux1/3
  [T_clt_2] -> Mux1/1
  Tank volume/1 -> Mixing/Mass factor - empirical/1
  [W_clt_1] -> Product5/1
  [p_clt_1] -> Sum/1
  [T_clt_1] -> Subtract/1
  [W_clt_1] -> Product1/2
  Subtract/1 -> Product1/1
  Integrator/1 -> [T_clt_2], Subtract/2
  Coolant density/1 -> Product5/2
  Mixing/Mass factor - empirical/1 -> Product/1
  Product/1 -> Divide/2
  Product1/1 -> Divide/1
  connector inlet area/1 -> Product3/2
  Sum/1 -> [p_clt_2]
  Product5/1 -> Product3/1
  Divide/1 -> Integrator/1
  F0014_tankPressureDrop.m/1 -> Sum/2
  Product3/1 -> F0014_tankPressureDrop.m/1  "v"
  Coolant density1/1 -> Product/2

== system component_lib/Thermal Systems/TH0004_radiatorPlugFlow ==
  CL: (T1,p1,W1) : Inport
  Demux1 : Demux  Outputs=3
  F0014_coreFlowDelay.m : base_lib/F0014_titanXradiator/F0014_coreFlowDelay.m  SystemSampleTime=-1  VariantActivationTime=update diagram  Latency=0  AutoFrameSizeCalculation=off
  Mux1 : Mux  Inputs=3
  Saturation1 : Saturate  UpperLimit=inf  LowerLimit=1e-5
  Variable Transport Delay1 : VariableTransportDelay  VariableDelayType=Variable transport delay  MaximumDelay=20  InitialOutput=T_0  MaximumPoints=10240  TransDelayFeedthrough=on
  CL: (T2,p2,W2) : Outport
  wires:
  F0014_coreFlowDelay.m/1 -> Variable Transport Delay1/2
  Variable Transport Delay1/1 -> Mux1/1
  CL: (T1,p1,W1)/1 -> Demux1/1
  Demux1/3 -> Saturation1/1
  Demux1/2 -> [p_clt_1]
  Demux1/1 -> Variable Transport Delay1/1
  [p_clt_1] -> Mux1/2
  Mux1/1 -> CL: (T2,p2,W2)/1
  Saturation1/1 -> Mux1/3, F0014_coreFlowDelay.m/1

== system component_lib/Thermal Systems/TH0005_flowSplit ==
  A (T1,p1,W1) : Inport
  split [-] : Inport  Port=2
  Demux1 : Demux  Outputs=3
  Mux1 : Mux  Inputs=3
  Mux2 : Mux  Inputs=3
  Product : Product
  Sum : Sum  Inputs=-+|
  B (T2,p2,W2) : Outport
  " C (T3,p3,W3)" : Outport  Port=2
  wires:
  Product/1 -> Mux1/3, Sum/1
  A (T1,p1,W1)/1 -> Demux1/1
  Demux1/3 -> Sum/2, Product/1
  Mux1/1 -> B (T2,p2,W2)/1
  split [-]/1 -> Product/2
  Mux2/1 -> " C (T3,p3,W3)"/1
  Sum/1 -> Mux2/3
  Demux1/1 -> [T_1]
  Demux1/2 -> Mux2/2, Mux1/2
  [T_1] -> Mux1/1
  [T_1] -> Mux2/1

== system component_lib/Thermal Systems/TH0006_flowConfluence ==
  note: Average pressure
  B (T1,p1,W1) : Inport
  C (T2,p2,W2) : Inport  Port=2
  Constant : Constant
  Demux1 : Demux  Outputs=3
  Demux2 : Demux  Outputs=3
  Gain : Gain  Gain=gain
  Gain1 : Gain  Gain=1/2
  Integrator Limited : Integrator  InitialCondition=0.5  LimitOutput=on  UpperSaturationLimit=1  LowerSaturationLimit=0
  Mux1 : Mux  Inputs=3
  Product : Product
  Product1 : Product
  Sum : Sum  Inputs=|+-
  Sum1 : Sum  Inputs=|++
  Sum2 : Sum  Inputs=++|
  Sum3 : Sum  Inputs=-+|
  Sum4 : Sum  Inputs=|++
  A (T3,p3,W3) : Outport
  split [-] : Outport  Port=2
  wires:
  B (T1,p1,W1)/1 -> Demux1/1
  Mux1/1 -> A (T3,p3,W3)/1
  C (T2,p2,W2)/1 -> Demux2/1
  Sum/1 -> Gain/1
  Gain/1 -> Integrator Limited/1
  Integrator Limited/1 -> split [-]/1, Product/2, Sum3/1
  Demux1/1 -> [T_11]
  Demux2/1 -> [T_12]
  Demux1/3 -> Sum1/1
  Sum1/1 -> Mux1/3
  Demux2/3 -> Sum1/2
  Demux1/2 -> [p_11]
  Demux2/2 -> [p_12]
  [p_11] -> Sum/1
  [p_12] -> Sum/2
  [T_11] -> Product/1
  Product/1 -> Sum2/1
  Product1/1 -> Sum2/2
  Sum2/1 -> Mux1/1
  Constant/1 -> Sum3/2
  [p_11] -> Sum4/1
  Sum4/1 -> Gain1/1
  [p_12] -> Sum4/2
  Gain1/1 -> Mux1/2
  Sum3/1 -> Product1/1
  [T_12] -> Product1/2

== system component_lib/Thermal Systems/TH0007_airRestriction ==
  AIR: (T1,p1,W1) : Inport
  Demux1 : Demux  Outputs=3
  F0014_restrictionPressureDrop.m : base_lib/F0014_titanXradiator/F0014_restrictionPressureDrop.m  SystemSampleTime=-1  VariantActivationTime=update diagram  Latency=0  AutoFrameSizeCalculation=off
  Mux1 : Mux  Inputs=3
  Sum : Sum  Inputs=-+|
  AIR: (T2,p2,W2) : Outport
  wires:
  Mux1/1 -> AIR: (T2,p2,W2)/1
  AIR: (T1,p1,W1)/1 -> Demux1/1
  Demux1/3 -> Mux1/3, F0014_restrictionPressureDrop.m/3
  Demux1/1 -> F0014_restrictionPressureDrop.m/1, Mux1/1
  F0014_restrictionPressureDrop.m/1 -> Sum/1
  Sum/1 -> Mux1/2
  Demux1/2 -> F0014_restrictionPressureDrop.m/2, Sum/2

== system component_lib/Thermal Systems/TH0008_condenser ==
  AIR: (T1,p1,W1) : Inport
  Q [J/s] : Inport  Port=2
  AIrCp : Constant  Value=par.cp_air
  Demux1 : Demux  Outputs=3
  F0014_condenserPressureDrop.m : base_lib/F0014_titanXradiator/F0014_condenserPressureDrop.m  SystemSampleTime=-1  VariantActivationTime=update diagram  Latency=0  AutoFrameSizeCalculation=off
  Mux1 : Mux  Inputs=3
  Product3 : Product  Inputs=*//
  Saturation : Saturate  UpperLimit=inf  LowerLimit=0.001
  Saturation1 : Saturate  UpperLimit=373  LowerLimit=0
  Sum : Sum  Inputs=|+-
  Sum1 : Sum  Inputs=++|
  AIR: (T2,p2,W2) : Outport
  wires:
  AIR: (T1,p1,W1)/1 -> Demux1/1
  Mux1/1 -> AIR: (T2,p2,W2)/1
  Q [J/s]/1 -> Product3/1
  AIrCp/1 -> Product3/3
  Product3/1 -> Sum1/2  "dT"
  Demux1/1 -> [T_1]
  Saturation/1 -> Product3/2
  Demux1/3 -> Mux1/3, F0014_condenserPressureDrop.m/3, Saturation/1
  Sum1/1 -> Saturation1/1
  Saturation1/1 -> Mux1/1
  Demux1/2 -> [p_1]
  [p_1] -> F0014_condenserPressureDrop.m/2
  [T_1] -> F0014_condenserPressureDrop.m/1
  [p_1] -> Sum/1
  Sum/1 -> Mux1/2
  F0014_condenserPressureDrop.m/1 -> Sum/2
  [T_1] -> Sum1/1

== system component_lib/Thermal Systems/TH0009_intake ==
  AIR: (T1,p1,W1) : Inport
  v [m/s] : Inport  Port=2
  Demux1 : Demux  Outputs=3
  F0014_intakePressureIncrease.m : base_lib/F0014_titanXradiator/F0014_intakePressureIncrease.m  SystemSampleTime=-1  VariantActivationTime=update diagram  Latency=0  AutoFrameSizeCalculation=off
  Mux1 : Mux  Inputs=3
  Saturation : Saturate  UpperLimit=inf  LowerLimit=0
  Sum : Sum  Inputs=++|
  AIR: (T2,p2,W2) : Outport
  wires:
  Mux1/1 -> AIR: (T2,p2,W2)/1
  AIR: (T1,p1,W1)/1 -> Demux1/1
  Sum/1 -> Mux1/2
  Demux1/2 -> Sum/2, F0014_intakePressureIncrease.m/2
  F0014_intakePressureIncrease.m/1 -> Sum/1
  Demux1/3 -> Mux1/3
  Demux1/1 -> Mux1/1, F0014_intakePressureIncrease.m/1
  v [m/s]/1 -> Saturation/1
  Saturation/1 -> F0014_intakePressureIncrease.m/3

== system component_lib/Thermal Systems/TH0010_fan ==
  note: Density
  AIR: (T1,p1,W1) : Inport
  rel_speed [-] : Inport  Port=2
  Constant : Constant  Value=286
  Constant1 : Constant  Value=par.n_fan
  Constant2 : Constant  Value=par.dp0
  Constant3 : Constant  Value=3
  Constant4 : Constant  Value=par.P_nom
  Constant5 : Constant  Value=par.n_fan
  Demux1 : Demux  Outputs=3
  Divide : Product  Inputs=*//
  Divide1 : Product  Inputs=*//
  Divide2 : Product  Inputs=*/
  F0014_fanCurve.m : base_lib/F0014_titanXradiator/F0014_fanCurve.m  SystemSampleTime=-1  VariantActivationTime=update diagram  Latency=0  AutoFrameSizeCalculation=off
  Math Function : Math  Operator=square
  Math Function1 : Math  Operator=pow
  Mux : Mux  Inputs=3
  Product : Product
  Product1 : Product
  Product2 : Product  Inputs=3
  Ref. density : Constant  Value=1.18
  Sum : Sum  Inputs=|++
  Transfer Fcn : TransferFcn  Denominator=[0.1 1]
  AIR: (T2,p2,W2) : Outport
  P_fan [J/s] : Outport  Port=2
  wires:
  AIR: (T1,p1,W1)/1 -> Demux1/1
  Mux/1 -> AIR: (T2,p2,W2)/1
  Demux1/3 -> Mux/3, Divide/1
  Demux1/1 -> Mux/1, [T_1]
  [T_1] -> Divide1/2
  Constant/1 -> Divide1/3
  Divide1/1 -> Divide2/1, Divide/3
  Constant1/1 -> Divide/2
  Math Function/1 -> Product/1
  Constant2/1 -> Product/2
  Divide/1 -> F0014_fanCurve.m/1
  Product/1 -> F0014_fanCurve.m/2
  F0014_fanCurve.m/1 -> Product1/1
  Ref. density/1 -> Divide2/2
  Divide2/1 -> Product1/2
  Demux1/2 -> [p_1], Sum/1
  Product1/1 -> Sum/2
  Sum/1 -> Mux/2
  [p_1] -> Divide1/1
  Transfer Fcn/1 -> Math Function/1, Math Function1/1
  rel_speed [-]/1 -> Transfer Fcn/1
  Constant3/1 -> Math Function1/2
  Math Function1/1 -> Product2/1
  Constant4/1 -> Product2/2
  Product2/1 -> P_fan [J/s]/1
  Constant5/1 -> Product2/3

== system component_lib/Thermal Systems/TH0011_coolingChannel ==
  T_w [K] : Inport
  CL: (T1,p1,W1) : Inport  Port=2
  Demux : Demux  Outputs=3
  F0017_Nusselt.m : base_lib/F0017_channelCooling/F0017_Nusselt.m  SystemSampleTime=-1  VariantActivationTime=update diagram  Latency=0  AutoFrameSizeCalculation=off
  F0017_Prandtl.m : base_lib/F0017_channelCooling/F0017_Prandtl.m  SystemSampleTime=-1  VariantActivationTime=update diagram  Latency=0  AutoFrameSizeCalculation=off
  F0017_Reynolds.m : base_lib/F0017_channelCooling/F0017_Reynolds.m  SystemSampleTime=-1  VariantActivationTime=update diagram  Latency=0  AutoFrameSizeCalculation=off
  F0017_heatTransfer.m : base_lib/F0017_channelCooling/F0017_heatTransfer.m  SystemSampleTime=-1  VariantActivationTime=update diagram  Latency=0  AutoFrameSizeCalculation=off
  F0017_pressureDrop.m : base_lib/F0017_channelCooling/F0017_pressureDrop.m  SystemSampleTime=-1  VariantActivationTime=update diagram  Latency=0  AutoFrameSizeCalculation=off
  F0017_velocity.m : base_lib/F0017_channelCooling/F0017_velocity.m  SystemSampleTime=-1  VariantActivationTime=update diagram  Latency=0  AutoFrameSizeCalculation=off
  Gain : Gain  Gain=1/n_ch
  Gain1 : Gain  Gain=n_ch
  Gain2 : Gain  Gain=n_ch
  Mux : Mux  Inputs=3
  Sum : Sum  Inputs=-+|
  Q [J/s] : Outport
  CL: (T2,p2,W2) : Outport  Port=2
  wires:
  CL: (T1,p1,W1)/1 -> Demux/1
  Mux/1 -> CL: (T2,p2,W2)/1
  F0017_velocity.m/1 -> F0017_Reynolds.m/1, F0017_pressureDrop.m/1
  F0017_Reynolds.m/1 -> F0017_pressureDrop.m/2, F0017_Nusselt.m/1
  F0017_Prandtl.m/1 -> F0017_Nusselt.m/2
  Demux/1 -> F0017_heatTransfer.m/1
  T_w [K]/1 -> F0017_heatTransfer.m/2
  F0017_Nusselt.m/1 -> F0017_heatTransfer.m/3
  Sum/1 -> [p_2]
  [p_2] -> Mux/2
  Demux/2 -> Sum/2
  Demux/3 -> Gain/1
  F0017_pressureDrop.m/1 -> Sum/1
  F0017_heatTransfer.m/1 -> Gain2/1
  F0017_heatTransfer.m/2 -> Mux/1
  Gain/1 -> F0017_velocity.m/1, Gain1/1, F0017_heatTransfer.m/4
  Gain1/1 -> Mux/3
  Gain2/1 -> Q [J/s]/1

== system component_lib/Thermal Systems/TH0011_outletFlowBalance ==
  AIR: (T1,p1,W1) : Inport
  p_amb [Pa] : Inport  Port=2
  Demux : Demux  Outputs=3
  Gain : Gain  Gain=gain
  Integrator Limited : Integrator  LimitOutput=on  LowerSaturationLimit=0
  Sum : Sum  Inputs=|+-
  Terminator : Terminator
  Terminator1 : Terminator
  W_inlet [kg/s] : Outport
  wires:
  AIR: (T1,p1,W1)/1 -> Demux/1
  Demux/2 -> Sum/1
  p_amb [Pa]/1 -> Sum/2
  Sum/1 -> Gain/1
  Gain/1 -> Integrator Limited/1
  Integrator Limited/1 -> W_inlet [kg/s]/1
  Demux/1 -> Terminator/1
  Demux/3 -> Terminator1/1

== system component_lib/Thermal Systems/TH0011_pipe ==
  CL: (T1,p1,W1) : Inport
  Constant : Constant  Value=par.L
  Demux : Demux  Outputs=3
  Divide : Product  Inputs=*/
  F0017_Reynolds.m : base_lib/F0017_channelCooling/F0017_Reynolds.m  SystemSampleTime=-1  VariantActivationTime=update diagram  Latency=0  AutoFrameSizeCalculation=off
  F0017_pressureDrop.m : base_lib/F0017_channelCooling/F0017_pressureDrop.m  SystemSampleTime=-1  VariantActivationTime=update diagram  Latency=0  AutoFrameSizeCalculation=off
  F0017_velocity.m : base_lib/F0017_channelCooling/F0017_velocity.m  SystemSampleTime=-1  VariantActivationTime=update diagram  Latency=0  AutoFrameSizeCalculation=off
  Mux : Mux  Inputs=3
  Saturation : Saturate  UpperLimit=10  LowerLimit=0
  Saturation1 : Saturate  UpperLimit=inf  LowerLimit=1e4
  Sum : Sum  Inputs=|+-
  Variable Transport Delay : VariableTransportDelay  VariableDelayType=Variable transport delay  MaximumDelay=10  InitialOutput=T_0
  CL: (T2,p2,W2) : Outport
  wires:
  CL: (T1,p1,W1)/1 -> Demux/1
  Constant/1 -> Divide/1
  F0017_velocity.m/1 -> F0017_Reynolds.m/1, Divide/2, F0017_pressureDrop.m/1
  Divide/1 -> Saturation/1
  Demux/1 -> Variable Transport Delay/1
  F0017_Reynolds.m/1 -> F0017_pressureDrop.m/2
  F0017_pressureDrop.m/1 -> Sum/2
  Saturation/1 -> Variable Transport Delay/2
  Variable Transport Delay/1 -> Mux/1
  Sum/1 -> Saturation1/1
  Mux/1 -> CL: (T2,p2,W2)/1
  Demux/3 -> Mux/3, F0017_velocity.m/1
  Demux/2 -> Sum/1
  Saturation1/1 -> Mux/2

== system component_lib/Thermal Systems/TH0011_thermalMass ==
  dQ [J/s] : Inport
  Constant : Constant  Value=m
  Constant1 : Constant  Value=cp
  Integrator : Integrator  InitialCondition=T_0
  Product : Product  Inputs=*//
  T [K] : Outport
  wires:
  Integrator/1 -> T [K]/1
  Product/1 -> Integrator/1
  dQ [J/s]/1 -> Product/1
  Constant/1 -> Product/2
  Constant1/1 -> Product/3

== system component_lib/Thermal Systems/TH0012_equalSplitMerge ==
  note: merge/distribute flow
  CL: (T1,p1,W1) : Inport
  Demux : Demux  Outputs=3
  Gain : Gain  Gain=n
  Mux : Mux  Inputs=3
  CL: (T2,p2,W2) : Outport
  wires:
  CL: (T1,p1,W1)/1 -> Demux/1
  Demux/3 -> Gain/1
  Demux/1 -> Mux/1
  Gain/1 -> Mux/3
  Demux/2 -> Mux/2
  Mux/1 -> CL: (T2,p2,W2)/1

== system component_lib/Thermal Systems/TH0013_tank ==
  W_pump [kg/s] : Inport
  p2 [Pa] : Inport  Port=2
  CL: (T1,p1,W1) : Inport  Port=3
  Constant : Constant  Value=par.cv_clt
  Constant1 : Constant  Value=par.cv_clt
  Constant2 : Constant  Value=T0
  Demux : Demux  Outputs=3
  Divide : Product  Inputs=*//
  Divide1 : Product  Inputs=***
  F0017_temperatureToEnthalpy.m : base_lib/F0017_channelCooling/F0017_temperatureToEnthalpy.m  SystemSampleTime=-1  VariantActivationTime=update diagram  Latency=0  AutoFrameSizeCalculation=off
  F0017_temperatureToEnthalpy.m1 : base_lib/F0017_channelCooling/F0017_temperatureToEnthalpy.m  SystemSampleTime=-1  VariantActivationTime=update diagram  Latency=0  AutoFrameSizeCalculation=off
  Integrator : Integrator  InitialCondition=V .* par.rho_clt  LimitOutput=on  LowerSaturationLimit=1e-3
  Integrator1 : Integrator  InitialConditionSource=external  InitialCondition=293  LimitOutput=on  LowerSaturationLimit=1e-3
  Mux : Mux  Inputs=3
  Product : Product
  Product1 : Product
  Sum : Sum  Inputs=+|-
  Sum2 : Sum  Inputs=+--
  Sum3 : Sum  Inputs=|-+
  Terminator : Terminator
  CL: (T2,p2,W2) : Outport
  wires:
  CL: (T1,p1,W1)/1 -> Demux/1
  Mux/1 -> CL: (T2,p2,W2)/1
  Sum/1 -> Divide1/3, Integrator/1
  Demux/3 -> Product/2, Sum/1
  Integrator/1 -> Divide/3
  p2 [Pa]/1 -> Mux/2
  Demux/2 -> Terminator/1
  Demux/1 -> F0017_temperatureToEnthalpy.m/1, [T_1]
  F0017_temperatureToEnthalpy.m/1 -> Product/1
  F0017_temperatureToEnthalpy.m1/1 -> Product1/1
  Integrator1/1 -> F0017_temperatureToEnthalpy.m1/1, Sum3/2, Mux/1
  Constant/1 -> Divide/2
  W_pump [kg/s]/1 -> Product1/2, Mux/3, Sum/2
  [T_1] -> Sum3/1
  Sum3/1 -> Divide1/2
  Sum2/1 -> Divide/1
  Divide1/1 -> Sum2/2
  Divide/1 -> Integrator1/1
  Constant1/1 -> Divide1/1
  Product/1 -> Sum2/1
  Product1/1 -> Sum2/3
  Constant2/1 -> Integrator1/2

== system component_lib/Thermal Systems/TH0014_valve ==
  open [-] : Inport
  CL: (T1,p1,W1) : Inport  Port=2
  split [-] : Inport  Port=3
  Constant : Constant  Value=par.d
  Constant1 : Constant
  Constant2 : Constant
  Constant3 : Constant  Value=par.d
  Demux : Demux  Outputs=3
  F0017_incompressibleRestriction.m : base_lib/F0017_channelCooling/F0017_incompressibleRestriction.m  SystemSampleTime=-1  VariantActivationTime=update diagram  Latency=0  AutoFrameSizeCalculation=off
  F0017_incompressibleRestriction.m1 : base_lib/F0017_channelCooling/F0017_incompressibleRestriction.m  SystemSampleTime=-1  VariantActivationTime=update diagram  Latency=0  AutoFrameSizeCalculation=off
  Mux : Mux  Inputs=3
  Mux1 : Mux  Inputs=3
  Product{,1..3} (4 alike) : Product
  Saturation : Saturate  UpperLimit=1  LowerLimit=0
  Saturation1 : Saturate  UpperLimit=0.99  LowerLimit=0.01
  Sum : Sum  Inputs=-+|
  Sum1 : Sum  Inputs=-+|
  Sum2 : Sum  Inputs=|+-
  Sum3 : Sum  Inputs=|+-
  Transfer Fcn : TransferFcn  Denominator=[0.1 1]
  CL: (T2,p2,W2) : Outport
  CL: (T3,p3,W3) : Outport  Port=2
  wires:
  CL: (T1,p1,W1)/1 -> Demux/1
  Mux/1 -> CL: (T2,p2,W2)/1
  Saturation1/1 -> Sum/1, Product/1
  Constant1/1 -> Sum/2
  Sum/1 -> Product1/2
  Constant2/1 -> Sum1/2
  Product2/1 -> F0017_incompressibleRestriction.m/1, [W_21]
  Product3/1 -> F0017_incompressibleRestriction.m1/1, [W_20]
  Sum1/1 -> Product3/2
  Demux/3 -> Product3/1, Product2/1
  Mux1/1 -> CL: (T3,p3,W3)/1
  Sum2/1 -> Mux/2
  F0017_incompressibleRestriction.m/1 -> Sum2/2
  Demux/1 -> Mux1/1, Mux/1
  [W_20] -> Mux1/3
  Demux/2 -> [p_1]
  Sum3/1 -> Mux1/2
  [p_1] -> Sum3/1
  F0017_incompressibleRestriction.m1/1 -> Sum3/2
  [p_1] -> Sum2/1
  [W_21] -> Mux/3
  Saturation/1 -> Sum1/1, Product2/2
  split [-]/1 -> Saturation/1
  open [-]/1 -> Transfer Fcn/1
  Transfer Fcn/1 -> Saturation1/1
  Constant/1 -> Product/2
  Constant3/1 -> Product1/1
  Product/1 -> F0017_incompressibleRestriction.m/2
  Product1/1 -> F0017_incompressibleRestriction.m1/2

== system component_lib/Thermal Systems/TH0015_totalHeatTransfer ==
  Q [J/s] : Inport
  CL: (T1,p1,W1) : Inport  Port=2
  Constant : Constant  Value=par.cp_clt
  Demux : Demux  Outputs=3
  Mux : Mux  Inputs=3
  Product : Product  Inputs=*//
  Saturation : Saturate  UpperLimit=T_max  LowerLimit=T_min
  Sum : Sum  Inputs=++|
  CL: (T2,p2,W2) : Outport
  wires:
  CL: (T1,p1,W1)/1 -> Demux/1
  Mux/1 -> CL: (T2,p2,W2)/1
  Demux/3 -> Mux/3, Product/2
  Demux/2 -> Mux/2
  Q [J/s]/1 -> Product/1
  Constant/1 -> Product/3
  Demux/1 -> Sum/2
  Product/1 -> Sum/1
  Sum/1 -> Saturation/1
  Saturation/1 -> Mux/1
